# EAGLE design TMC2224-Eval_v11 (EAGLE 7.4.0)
CHECK_DATE: 24.01.14; DRAW_DATE: 27.01.14; PROJECT: DRV_Board_TMC261; REV: v1.0

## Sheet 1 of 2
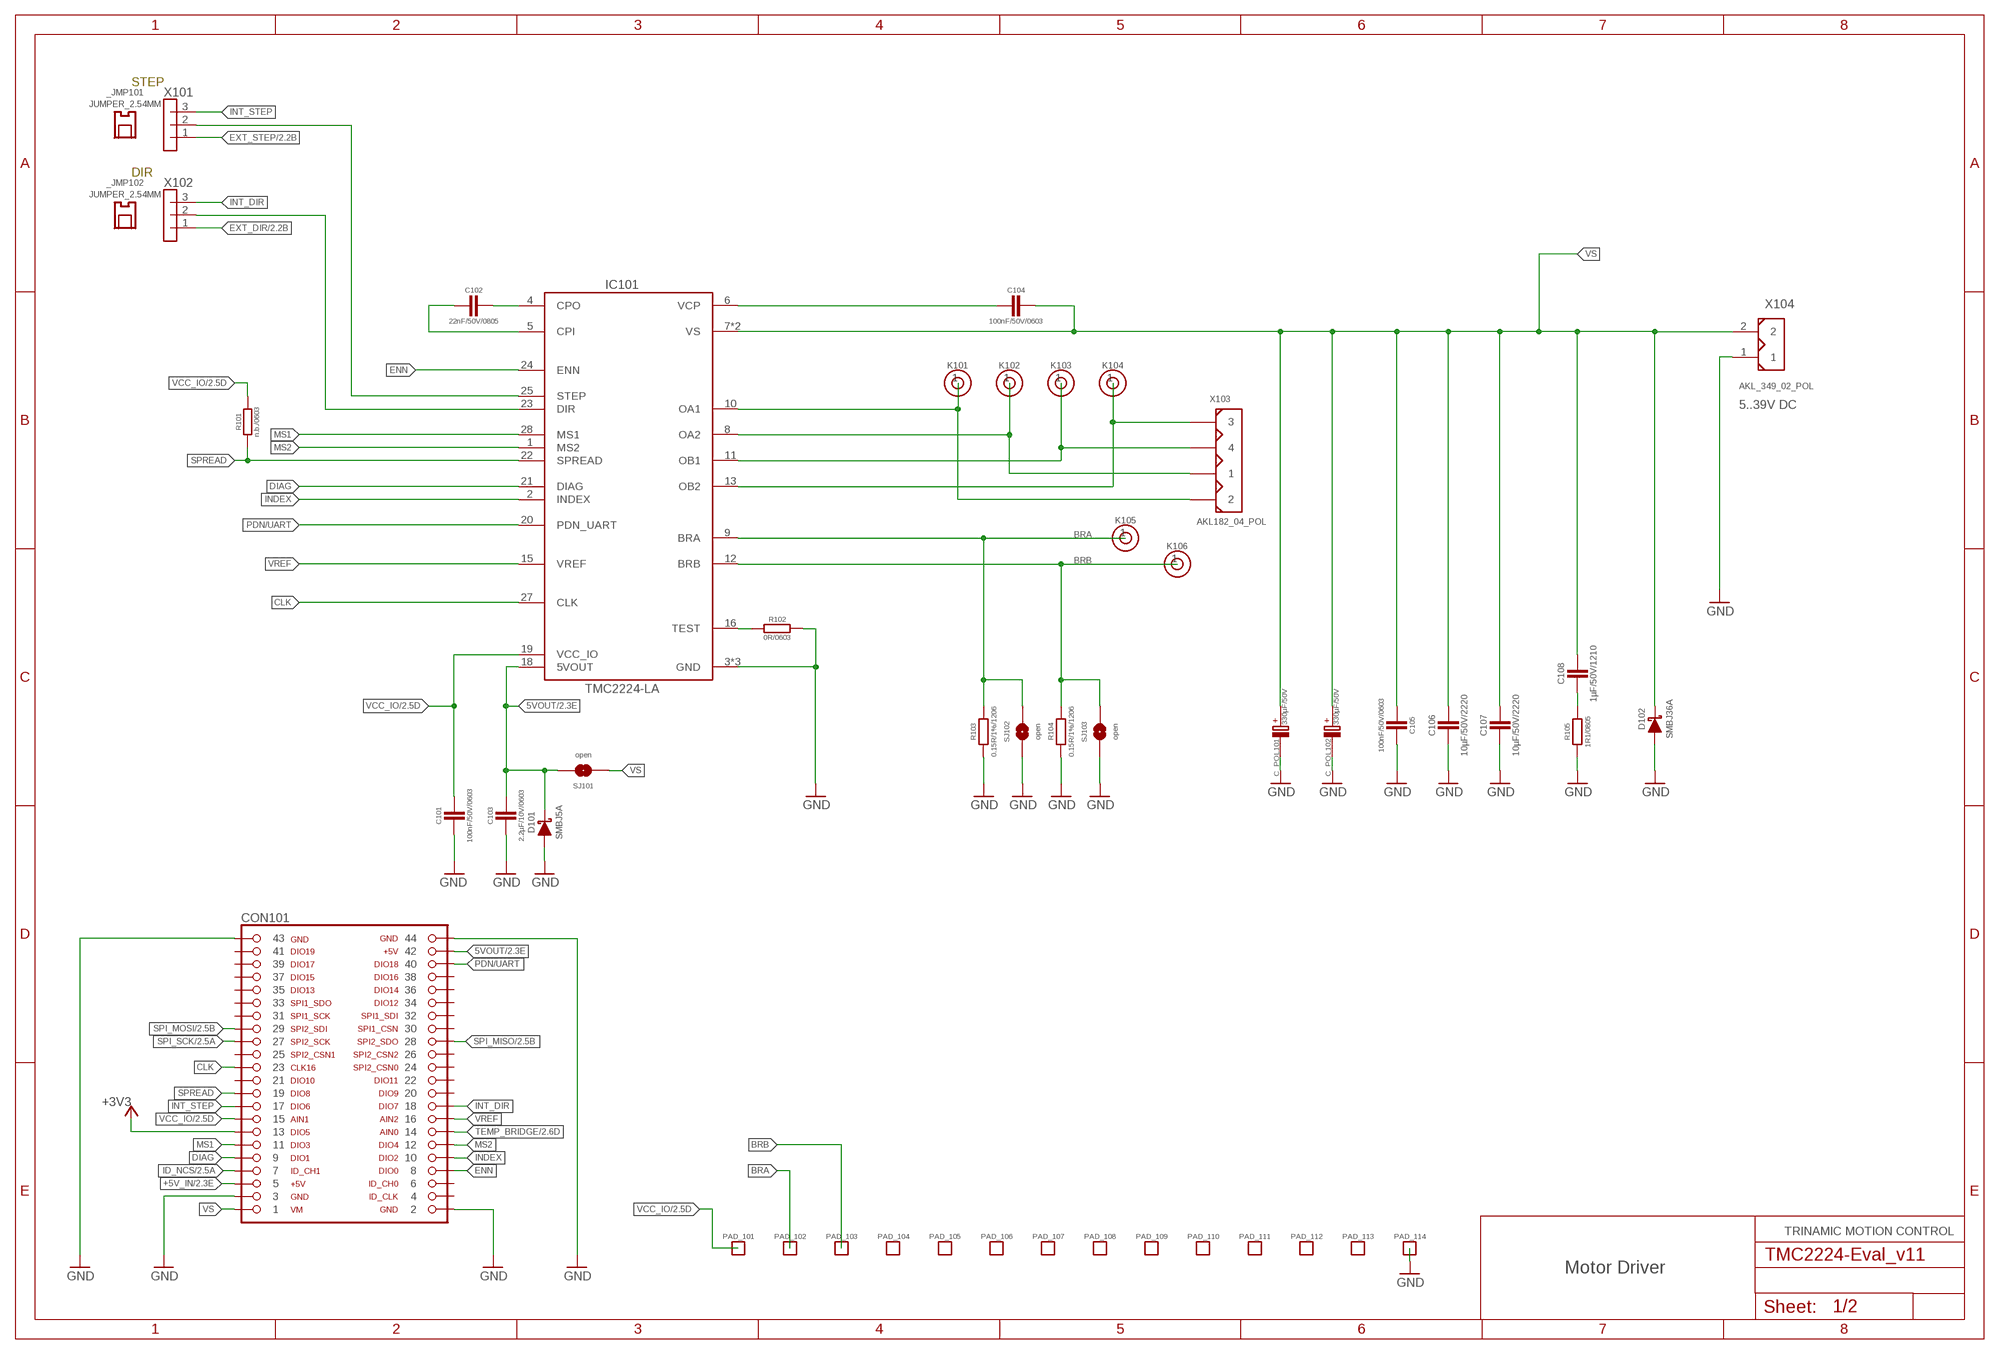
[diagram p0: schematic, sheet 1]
_JMP101 (JUMPER_2.54MM): ADGPN: 3044010200; DATASHEET: http://www.tme.eu/en/Document/d9e6fb6fc4dc34d59ba745016c42e7c7/jumper.pdf; MANUF-CODE-1: JUMPER-B; MANUFACTURER-1: Ninigi; PRICE: 0.11; SUPPLIER: TME; SUPPLIER-CODE: JUMPER-B
_JMP102 (JUMPER_2.54MM): ADGPN: 3044010200; DATASHEET: http://www.tme.eu/en/Document/d9e6fb6fc4dc34d59ba745016c42e7c7/jumper.pdf; MANUF-CODE-1: JUMPER-B; MANUFACTURER-1: Ninigi; PRICE: 0.11; SUPPLIER: TME; SUPPLIER-CODE: JUMPER-B

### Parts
C101  100nF/50V/0603  C0603  [_RC_0603]
C102  22nF/50V/0805  C0805  [_RC_0805]
C103  2.2µF/10V/0603  C0603  [_RC_0603]
C104  100nF/50V/0603  C0603  [_RC_0603]
C105  100nF/50V/0603  C0603  [_RC_0603]
C106  10µF/50V/2220  C2220  [C2220]
C107  10µF/50V/2220  C2220  [C2220]
C108  1µF/50V/1210  C1210  [C1210]
C_POL101  330µF/50V  C_POL5X10X17.5  [C_POL_RAD_THT_5X10]
C_POL102  330µF/50V  C_POL5X10X17.5  [C_POL_RAD_THT_5X10]
CON101  FEMALE_HEADER_SMD_2.54_44_PINSHORTPADS_HOLES  [FEMALE_HEADER_SMD_254_44_PIN_SHORTPADS_HOLES]
D101  SMBJ5A  SMBJ  [D_SMB]
D102  SMBJ36A  SMBJ48A  [D_SMB]
IC101  TMC2224-LA  [QFN28P]
K101  1PIN_1ROW  [1PIN_1ROW_THT]
K102  1PIN_1ROW  [1PIN_1ROW_THT]
K103  1PIN_1ROW  [1PIN_1ROW_THT]
K104  1PIN_1ROW  [1PIN_1ROW_THT]
K105  1PIN_1ROW  [1PIN_1ROW_THT]
K106  1PIN_1ROW  [1PIN_1ROW_THT]
PAD_101  PAD_ROUND  [PAD_R1.2]
PAD_102  PAD_ROUND  [PAD_R1.2]
PAD_103  PAD_ROUND  [PAD_R1.2]
PAD_104  PAD_ROUND  [PAD_R1.2]
PAD_105  PAD_ROUND  [PAD_R1.2]
PAD_106  PAD_ROUND  [PAD_R1.2]
PAD_107  PAD_ROUND  [PAD_R1.2]
PAD_108  PAD_ROUND  [PAD_R1.2]
PAD_109  PAD_ROUND  [PAD_R1.2]
PAD_110  PAD_ROUND  [PAD_R1.2]
PAD_111  PAD_ROUND  [PAD_R1.2]
PAD_112  PAD_ROUND  [PAD_R1.2]
PAD_113  PAD_ROUND  [PAD_R1.2]
PAD_114  PAD_ROUND  [PAD_R1.2]
R101  n.b./0603  0R/0603  [_RC_0603]
R102  0R/0603  [_RC_0603]
R103  0.15R/1%/1206  R1206  [_RC_1206]
R104  0.15R/1%/1206  R1206  [_RC_1206]
R105  1R1/0805  R0805  [_RC_0805]
SJ101  open  SJ  [_SJ_0402]
SJ102  open  SJ  [_SJ_0402]
SJ103  open  SJ  [_SJ_0402]
X101  3PIN_1ROWTHT  [3PIN_1ROM_2,54_THT]
X102  3PIN_1ROWTHT  [3PIN_1ROM_2,54_THT]
X103  AKL182_04_POL  [AKL169_04_POL]
X104  AKL_349_02_POL  [AKL349_02_POL]

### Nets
5VOUT: C103.P$1 CON101.42 D101.C IC101.18(5VOUT) SJ101.P$2 ; also sheet 2
+3V3: CON101.13 ; also sheet 2
+5V_IN: CON101.5 ; also sheet 2
BRA: IC101.9(BRA) K105.1 PAD_102.P$1 R103.P$2 SJ102.P$2
BRB: IC101.12(BRB) K106.1 PAD_103.P$1 R104.P$2 SJ103.P$2
CLK: CON101.23 IC101.27(CLK)
CPI: C102.P$2 IC101.5(CPI)
CPO: C102.P$1 IC101.4(CPO)
DIAG: CON101.9 IC101.21(DIAG)
DIR: IC101.23(DIR) X102.2
ENN: CON101.8 IC101.24(ENN)
EXT_DIR: X102.1 ; also sheet 2
EXT_STEP: X101.1 ; also sheet 2
GND: C101.P$2 C103.P$2 C105.P$2 C106.2 C107.2 C_POL101.- C_POL102.- CON101.2 CON101.3 CON101.43 CON101.44 D101.A D102.A IC101.3(GND) IC101.17(GND) IC101.PAD(GND) PAD_114.P$1 R102.P$2 R103.P$1 R104.P$1 R105.P$1 SJ102.P$1 SJ103.P$1 X104.1 ; also sheet 2
ID_NCS: CON101.7 ; also sheet 2
INDEX: CON101.10 IC101.2(INDEX)
INT_DIR: CON101.18 X102.3
INT_STEP: CON101.17 X101.3
MS1: CON101.11 IC101.28(MS1)
MS2: CON101.12 IC101.1(MS2)
N$2: C108.2 R105.P$2
OA1: IC101.10(OA1) K101.1 X103.1
OA2: IC101.8(OA2) K102.1 X103.2
OB1: IC101.11(OB1) K103.1 X103.3
OB2: IC101.13(OB2) K104.1 X103.4
PDN/UART: CON101.40 IC101.20(PDN_UART)
SPI_MISO: CON101.28 ; also sheet 2
SPI_MOSI: CON101.29 ; also sheet 2
SPI_SCK: CON101.27 ; also sheet 2
SPREAD: CON101.19 IC101.22(SPREAD) R101.P$1
STEP: IC101.25(STEP) X101.2
TEMP_BRIDGE: CON101.14 ; also sheet 2
TEST: IC101.16(TEST) R102.P$1
VCC_IO: C101.P$1 CON101.15 IC101.19(VCC_IO) PAD_101.P$1 R101.P$2 ; also sheet 2
VCP: C104.P$1 IC101.6(VCP)
VREF: CON101.16 IC101.15(VREF)
VS: C104.P$2 C105.P$1 C106.1 C107.1 C108.1 C_POL101.+ C_POL102.+ CON101.1 D102.C IC101.7(VS) IC101.14(VS) SJ101.P$1 X104.2
Unconnected: CON101.4 CON101.6 CON101.20 CON101.21 CON101.22 CON101.24 CON101.25 CON101.26 CON101.30 CON101.31 CON101.32 CON101.33 CON101.34 CON101.35 CON101.36 CON101.37 CON101.38 CON101.39 CON101.41 PAD_104.P$1 PAD_105.P$1 PAD_106.P$1 PAD_107.P$1 PAD_108.P$1 PAD_109.P$1 PAD_110.P$1 PAD_111.P$1 PAD_112.P$1 PAD_113.P$1

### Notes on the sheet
- STEP
- DIR
- 5..39V DC
- TRINAMIC MOTION CONTROL
- Motor Driver

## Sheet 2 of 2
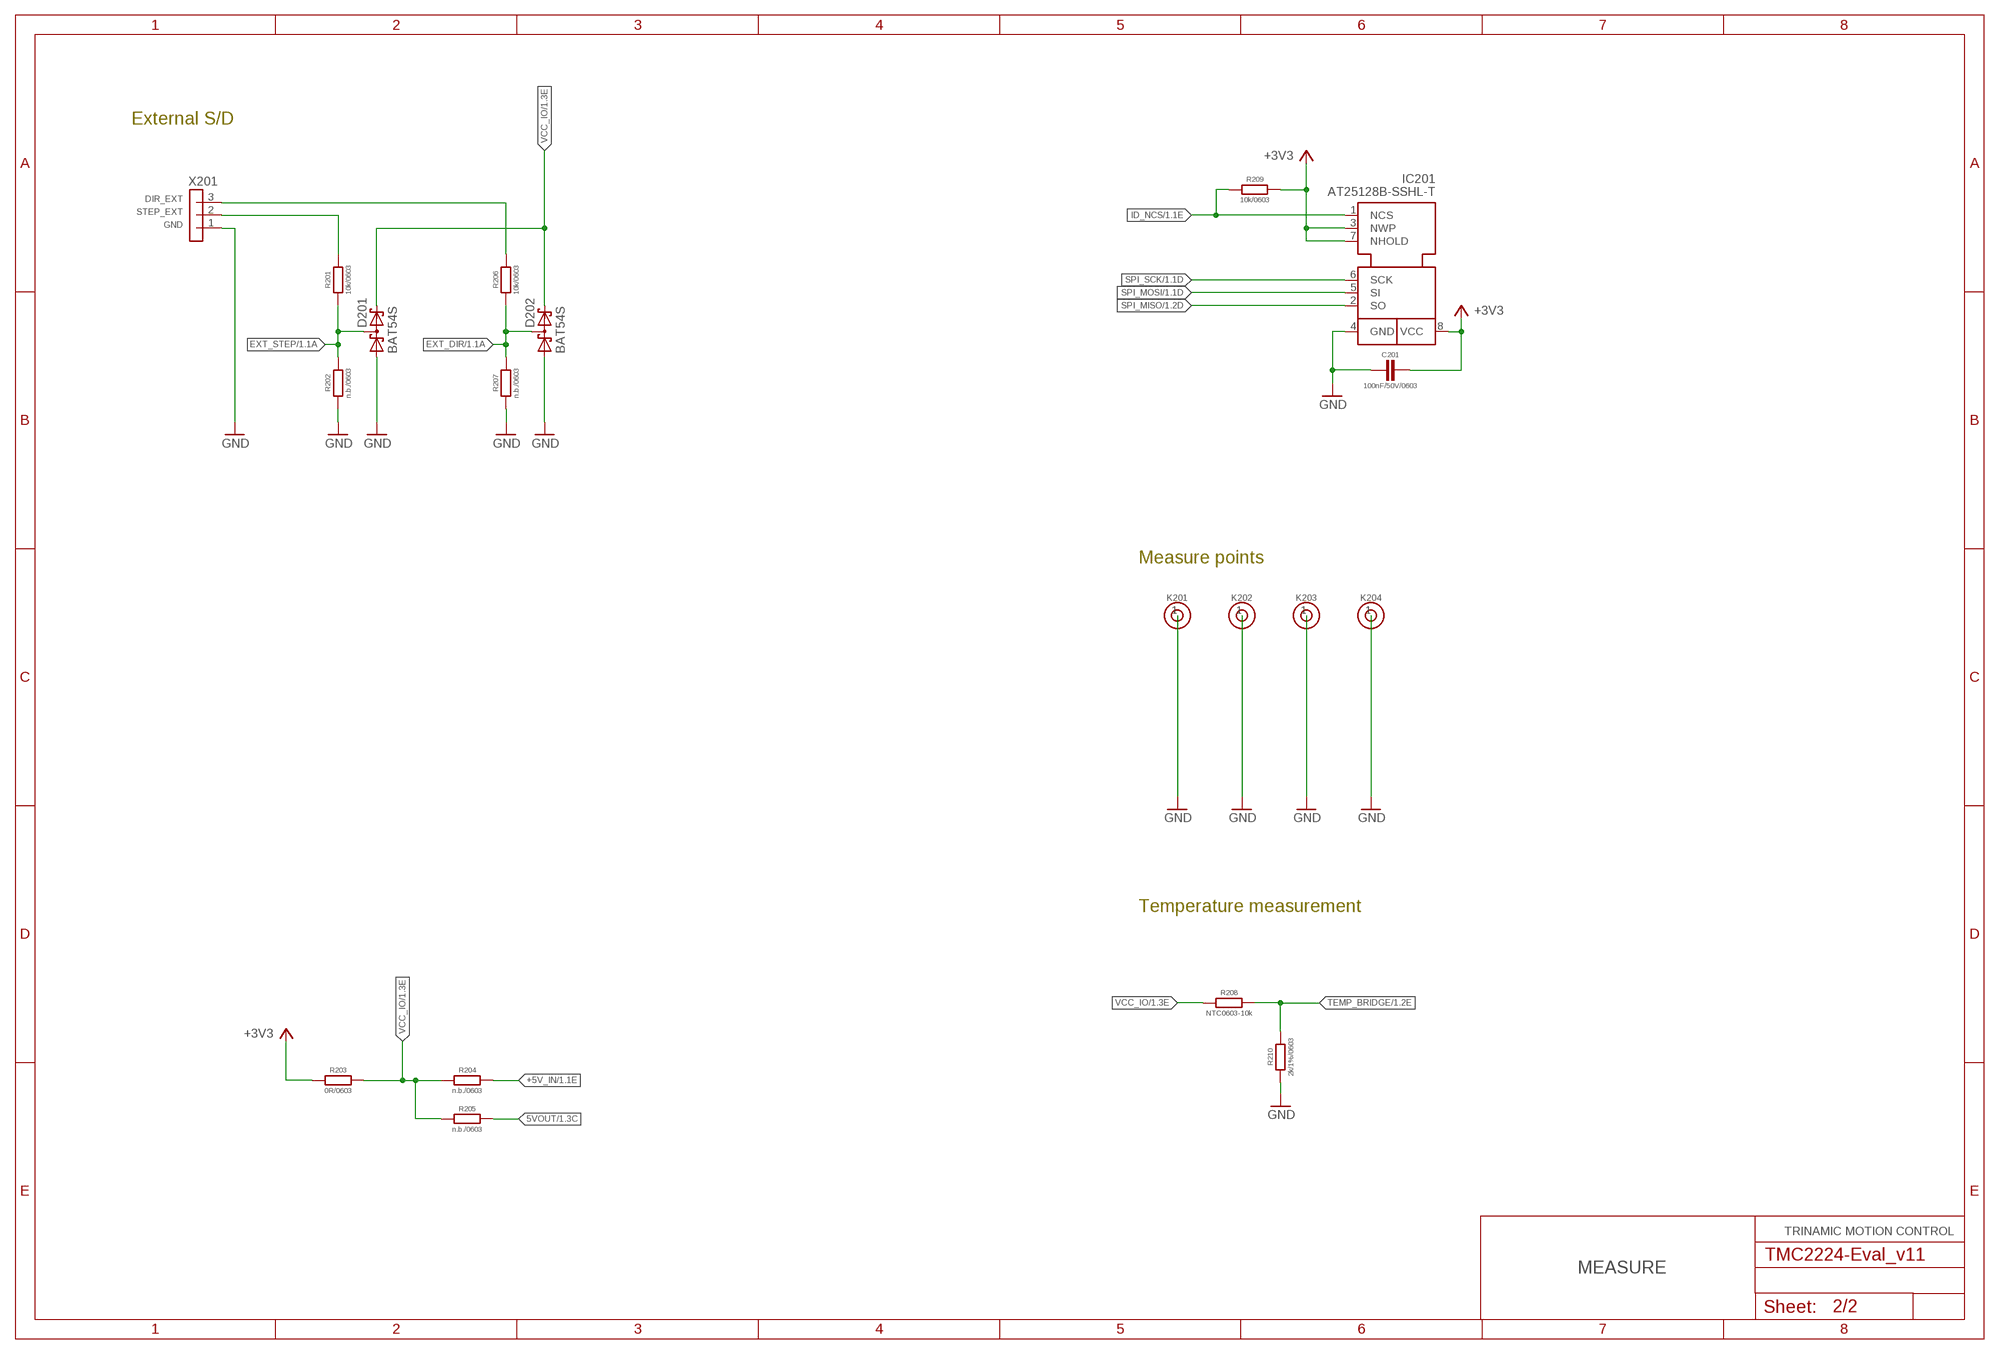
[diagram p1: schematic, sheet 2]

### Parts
C201  100nF/50V/0603  C0603  [_RC_0603]
D201  BAT54S  [SOT23]
D202  BAT54S  [SOT23]
IC201  AT25128B-SSHL-T  [SO8]
K201  1PIN_1ROW  [1PIN_1ROW_THT]
K202  1PIN_1ROW  [1PIN_1ROW_THT]
K203  1PIN_1ROW  [1PIN_1ROW_THT]
K204  1PIN_1ROW  [1PIN_1ROW_THT]
R201  10k/0603  R0603  [_RC_0603]
R202  n.b./0603  R0603  [_RC_0603]
R203  0R/0603  R0603  [_RC_0603]
R204  n.b./0603  R0603  [_RC_0603]
R205  n.b./0603  R0603  [_RC_0603]
R206  10k/0603  R0603  [_RC_0603]
R207  n.b./0603  R0603  [_RC_0603]
R208  NTC0603-10k  R0603  [_RC_0603]
R209  10k/0603  R0603  [_RC_0603]
R210  2k/1%/0603  R0603  [_RC_0603]
X201  3PIN_1ROWTHT  [3PIN_1ROM_2,54_THT]

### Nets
5VOUT: R205.P$2 ; also sheet 1
+3V3: C201.P$1 IC201.3(NWP) IC201.7(NHOLD) IC201.8(VCC) R203.P$1 R209.P$2 ; also sheet 1
+5V_IN: R204.P$2 ; also sheet 1
DIR_EXT: R206.P$2 X201.3
EXT_DIR: D202.3(C1A2) R206.P$1 R207.P$2 ; also sheet 1
EXT_STEP: D201.3(C1A2) R201.P$1 R202.P$2 ; also sheet 1
GND: C201.P$2 D201.1(A1) D202.1(A1) IC201.4(GND) K201.1 K202.1 K203.1 K204.1 R202.P$1 R207.P$1 R210.P$1 X201.1 ; also sheet 1
ID_NCS: IC201.1(NCS) R209.P$1 ; also sheet 1
SPI_MISO: IC201.2(SO) ; also sheet 1
SPI_MOSI: IC201.5(SI) ; also sheet 1
SPI_SCK: IC201.6(SCK) ; also sheet 1
STEP_EXT: R201.P$2 X201.2
TEMP_BRIDGE: R208.P$2 R210.P$2 ; also sheet 1
VCC_IO: D201.2(C2) D202.2(C2) R203.P$2 R204.P$1 R205.P$1 R208.P$1 ; also sheet 1

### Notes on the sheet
- External S/D
- Measure points
- Temperature measurement
- TRINAMIC MOTION CONTROL
- MEASURE

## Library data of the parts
C101-C105 C201 = TMC2208-Eval:C
C106 C107 = TMC2208-Eval:C*: Capacitor; OC_DIGIKEY: 445-7932-1-ND; SUPPLIER: DigiKey; SUPPLIER-CODE: 445-7932-1-ND
C108 = TMC2208-Eval:C*: Capacitor; OC_DIGIKEY: 1276-1811-1-ND; SUPPLIER: DigiKey; SUPPLIER-CODE: 1276-1811-1-ND
C_POL101 C_POL102 = TMC2208-Eval:C_POL; OC_DIGIKEY: 493-1343-ND; SUPPLIER: DigiKey; SUPPLIER-CODE: 493-1343-ND
CON101 = TMC2208-Eval:FEMALE_HEADER_SMD_2.54_44_PIN; SUPPLIER: MPE Garry; SUPPLIER-CODE: 098-3-044-1-NFX-YT0; SUPPLIER2: Samtec; SUPPLIER2-CODE: HLE-122-02-F-DV
D101 = TMC2208-Eval:SMBJ*: Surface Mount TRANSZORB Transient Voltage Suppressors 600W; MANUFACTURER: Bourns; OC_DIGIKEY: SMBJ5.0ABCT-ND; SUPPLIER: DigiKey; SUPPLIER-CODE: SMBJ5.0ABCT-ND
D102 = TMC2208-Eval:SMBJ*: Surface Mount TRANSZORB Transient Voltage Suppressors 600W; ADGPN: 4004048400; DATASHEET: http://www.bourns.com/data/global/pdfs/SMBJ.pdf; GEOMETRY_HEIGHT: 2.62mm; MANUFACTURER: Bourns; MANUFACTURER-CODE: SMBJ36A; OC_DIGIKEY: SMBJ36ABCT-ND; PRICE: 0,19; SUPPLIER: DigiKey; SUPPLIER-CODE: SMBJ36ABCT-ND
D201 D202 = TMC2208-Eval:BAT54S: SOT23, BAT54S, Double Schottky diode 30V 200mA Copied from diode.lbr and edited for Artec use 23-08-13 Pin connection corrected 2011-05-04 Source: Fairchild .. BAT54.pdf; ADGPN: 3522154300; DATASHEET: http://www.fairchildsemi.com/ds/BA/BAT54.pdf; MANUFACTURER: Fairchild; MANUFACTURER-CODE: BAT54S; OC_DIGIKEY: BAT54SFSCT-ND; PRICE: 0.12; SUPPLIER: DigiKey; SUPPLIER-CODE: BAT54SFSCT-ND
IC101 = TMC2224:TMC2224
IC201 = TMC2208-Eval:AT25128B; OC_DIGIKEY: AT25128B-SSHL-TCT-ND; SUPPLIER: DigiKey; SUPPLIER-CODE: AT25128B-SSHL-TCT-ND
K101-K106 K201-K204 = TMC2208-Eval:1PIN_1ROW
PAD_101-PAD_114 = TMC2208-Eval:PAD_ROUND
R101 R102 = TRI_R_0603:0R: Resistor (Jumper) 0603; MF: Panasonic; MPN: ERJ-3GEY0R00V; OC_DIGIKEY: P0.0GCT-ND; OR_SIMILAR: Yes; RATED_POWER: 1/10W
R103 R104 = TMC2208-Eval:R; OC_DIGIKEY: 408-1584-1-ND; SUPPLIER: DigiKey; SUPPLIER-CODE: 408-1584-1-ND
R105 = TMC2208-Eval:R; OC_DIGIKEY: RHM1.1KCT-ND; SUPPLIER-CODE: RHM1.1KCT-ND; SUPPLY: DigiKey
R201-R207 R209 R210 = TMC2208-Eval:R
R208 = TMC2208-Eval:R; OC_DIGIKEY: 445-174518-1-ND; SUPPLIER: DigiKey; SUPPLIER-CODE: 445-174518-1-ND
SJ101-SJ103 = TMC2208-Eval:SJ: SMD solder JUMPER
X101 X102 X201 = TMC2208-Eval:3PIN_1ROW
X103 = TMC2208-Eval:AKL182_04_POL; SUPPLIER: RIA CONNECT; SUPPLIER-CODE: 31182104; SUPPLIER2: Reichelt; SUPPLIER2-CODE: AKL 182-04
X104 = TMC2208-Eval:AKL_349_02_POL; SUPPLIER: RIA CONNECT; SUPPLIER-CODE: 31349102; SUPPLIER2: Reichelt; SUPPLIER2-CODE: AKL 349-02

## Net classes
0 default: clearance 0.2 mm
1 High Current: clearance 0.5 mm
2 VM: clearance 0.5 mm

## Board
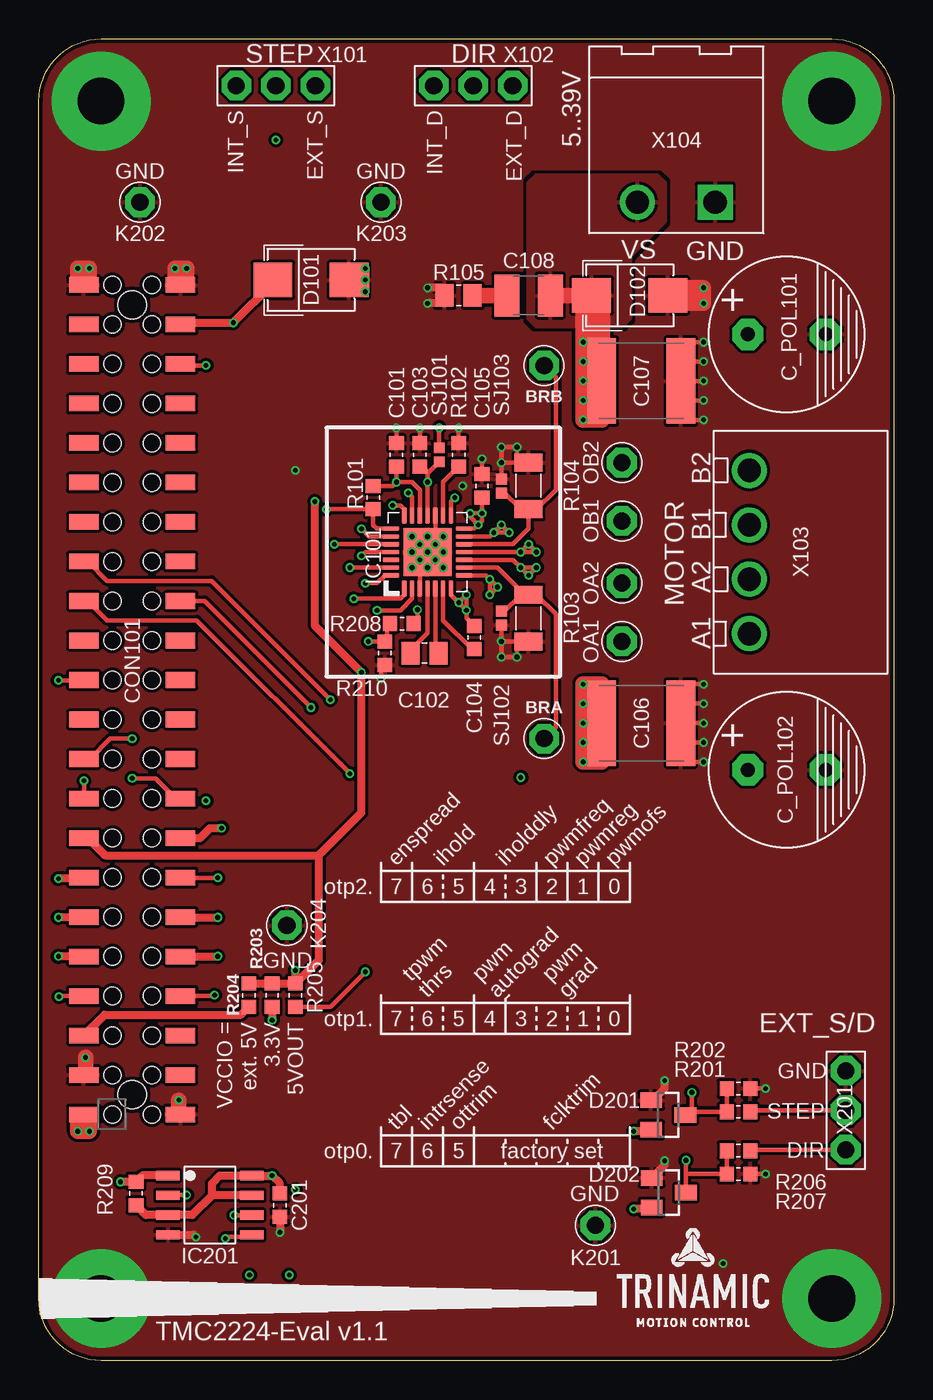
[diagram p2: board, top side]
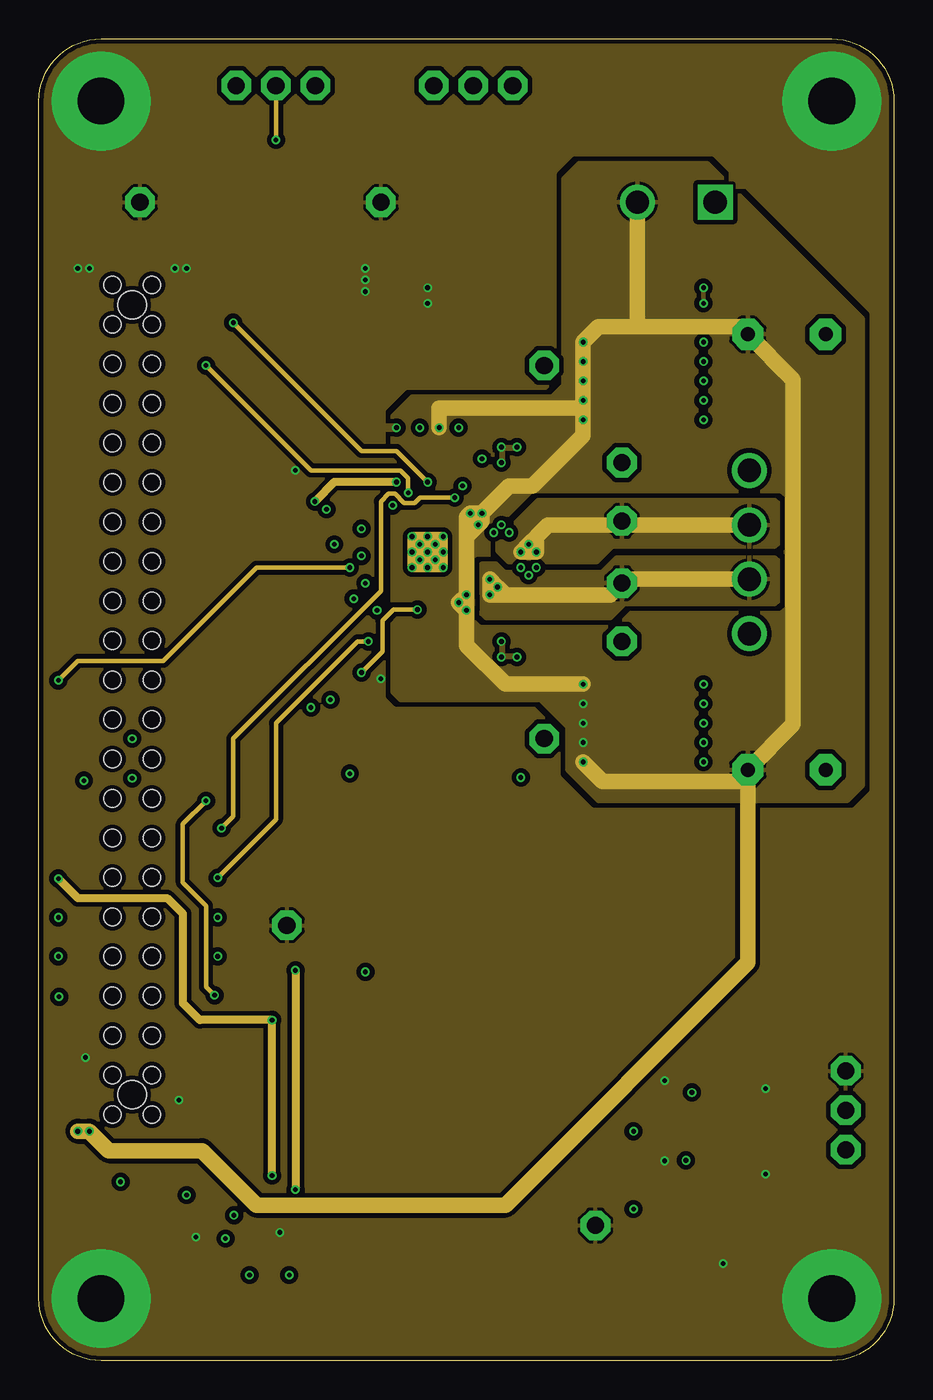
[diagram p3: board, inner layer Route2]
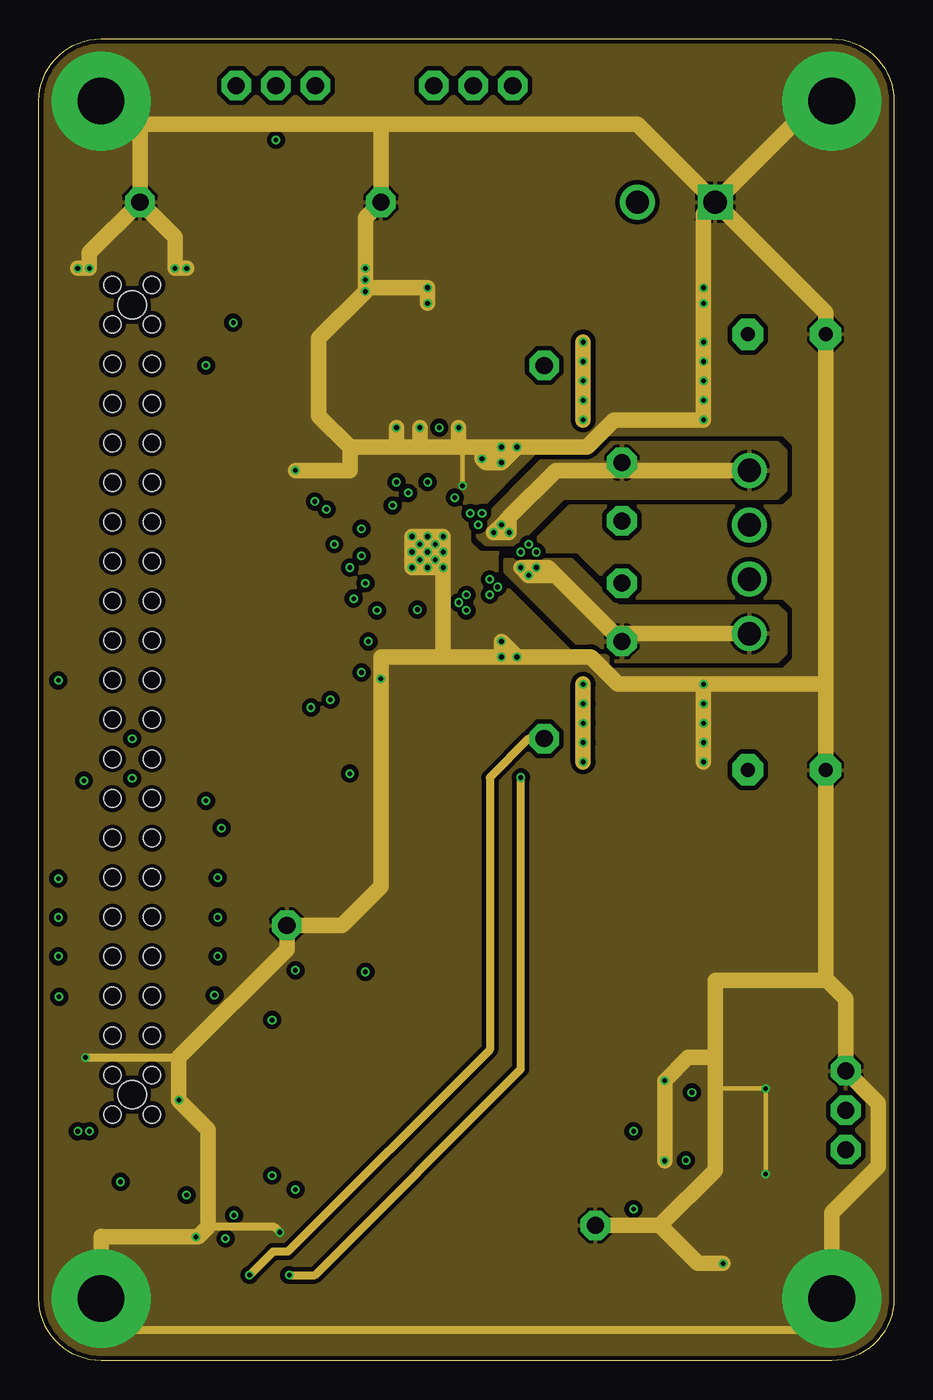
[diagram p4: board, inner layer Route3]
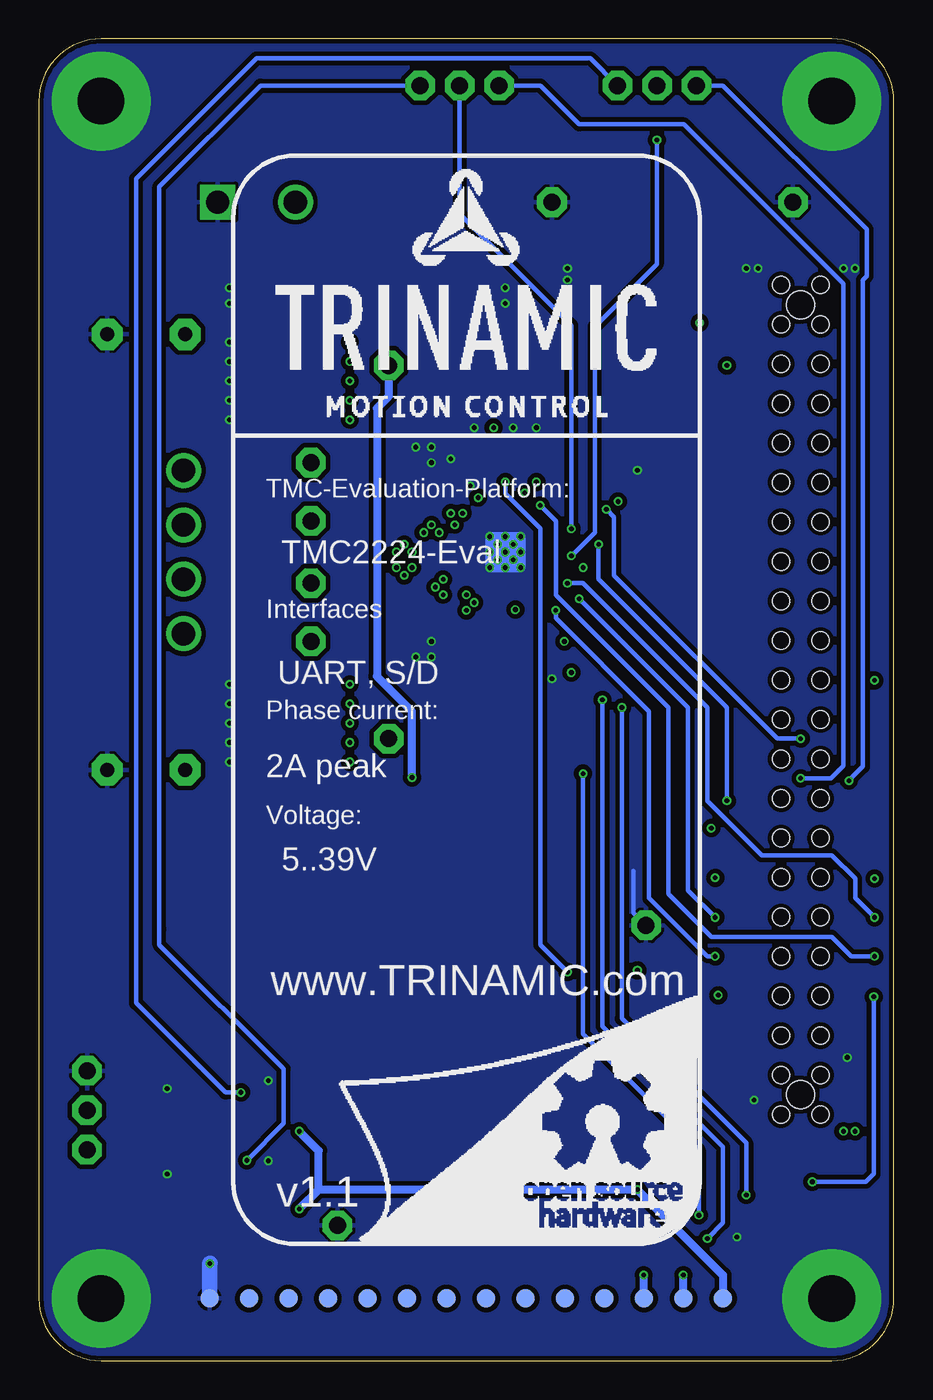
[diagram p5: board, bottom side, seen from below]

Size 55 x 85 mm. Coordinates in mm from the lower left corner, seen from the top.
Outline: 51,0 4,0 arc-90 0,4 0,81 arc-90 4,85 51,85 arc-90 55,81 55,4 arc-90 51,0
Copper layers (1+2*3+16): Top 0.018mm / dielectric 0.36mm / Route2 0.035mm / dielectric 0.71mm / Route3 0.035mm / dielectric 0.36mm / Bottom 0.018mm
Design rules "eC_4Layer_PClass6_BaseCopperO18-I35_eCDefault *": minimum track width 0.15mm, minimum drill 0.3mm, track to track 0.15mm, track to pad 0.15mm, pad to pad 0.15mm, via to via 0.15mm, smd to smd 0mil, copper to edge 0.25mm, drill to drill 0.33mm, minimum pad ring 0.175mm, minimum via ring 0.125mm, stop-mask expansion 0mil, vias tented up to drill 0.45mm, thermal gap 0.2mm

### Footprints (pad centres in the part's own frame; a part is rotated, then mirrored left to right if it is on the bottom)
_RC_0603 = smd 0.9 x 0.95: P$1 -0.75,0; P$2 0.75,0
_RC_0805 = smd 1.15 x 1.45: P$1 -0.9,0; P$2 0.9,0
C2220 = smd 1.85 x 5.5: 1 -2.55,0; 2 2.55,0
C1210 = smd 1.6 x 2.7: 1 -1.4,0; 2 1.4,0
C_POL_RAD_THT_5X10 = drill 0.9 pad 2 octagon: + 2.5,0; - -2.5,0
FEMALE_HEADER_SMD_254_44_PIN_SHORTPADS_HOLES = smd 1 x 1.9: 1 -26.67,3.11; 2 -26.67,-3.11; 3 -24.13,3.11; 4 -24.13,-3.11; 5 -21.59,3.11; 6 -21.59,-3.11; 7 -19.05,3.11; 8 -19.05,-3.11; 9 -16.51,3.11; 10 -16.51,-3.11; 11 -13.97,3.11; 12 -13.97,-3.11; 13 -11.43,3.11; 14 -11.43,-3.11; 15 -8.89,3.11; 16 -8.89,-3.11; 17 -6.35,3.11; 18 -6.35,-3.11; 19 -3.81,3.11; 20 -3.81,-3.11; 21 -1.27,3.11; 22 -1.27,-3.11; 23 1.27,3.11; 24 1.27,-3.11; 25 3.81,3.11; 26 3.81,-3.11; 27 6.35,3.11; 28 6.35,-3.11; 29 8.89,3.11; 30 8.89,-3.11; 31 11.43,3.11; 32 11.43,-3.11; 33 13.97,3.11; 34 13.97,-3.11; 35 16.51,3.11; 36 16.51,-3.11; 37 19.05,3.11; 38 19.05,-3.11; 39 21.59,3.11; 40 21.59,-3.11; 41 24.13,3.11; 42 24.13,-3.11; 43 26.67,3.11; 44 26.67,-3.11 | hole 1.8: -25.4,0; 25.4,0 | hole 1.1: -26.67,1.27; -24.13,1.27; -21.59,1.27; -19.05,1.27; -16.51,1.27; -13.97,1.27; -11.43,1.27; -8.89,1.27; -6.35,1.27; -3.81,1.27; -1.27,1.27; 1.27,1.27; 3.81,1.27; 6.35,1.27; 8.89,1.27; 11.43,1.27; 13.97,1.27; 16.51,1.27; 19.05,1.27; 21.59,1.27; 24.13,1.27; 26.67,1.27; -26.67,-1.27; -24.13,-1.27; -21.59,-1.27; -19.05,-1.27; -16.51,-1.27; -13.97,-1.27; -11.43,-1.27; -8.89,-1.27; -6.35,-1.27; -3.81,-1.27; -1.27,-1.27; 1.27,-1.27; 3.81,-1.27; 6.35,-1.27; 8.89,-1.27; 11.43,-1.27; 13.97,-1.27; 16.51,-1.27; 19.05,-1.27; 21.59,-1.27; 24.13,-1.27; 26.67,-1.27
D_SMB = smd 2.5 x 2.2: A 2.45,0; C -2.45,0
SOT23 = smd 1 x 1.4: 1 -0.95,-1.1; 2 0.95,-1.1; 3 0,1.1
QFN28P = smd 1.05 x 0.3: 1 -2.35,1.5; 2 -2.35,1; 3 -2.35,0.5; 4 -2.35,0; 5 -2.35,-0.5; 6 -2.35,-1; 7 -2.35,-1.5; 15 2.35,-1.5; 16 2.35,-1; 17 2.35,-0.5; 18 2.35,0; 19 2.35,0.5; 20 2.35,1; 21 2.35,1.5 | smd 0.3 x 1.05: 8 -1.5,-2.35; 9 -1,-2.35; 10 -0.5,-2.35; 11 0,-2.35; 12 0.5,-2.35; 13 1,-2.35; 14 1.5,-2.35; 22 1.5,2.35; 23 1,2.35; 24 0.5,2.35; 25 0,2.35; 26 -0.5,2.35; 27 -1,2.35; 28 -1.5,2.35 | smd 3.1 x 3.1: PAD 0,0
SO8 = smd 1.5 x 0.6: 1 -2.7,1.905; 2 -2.7,0.635; 3 -2.7,-0.635; 4 -2.7,-1.905; 5 2.7,-1.905; 6 2.7,-0.635; 7 2.7,0.635; 8 2.7,1.905
1PIN_1ROW_THT = drill 1.1 pad 1.9 octagon: 1 0,0
PAD_R1.2 = smd 1.2 x 1.2: P$1 0,0
_RC_1206 = smd 1.15 x 1.8: P$1 -1.5,0; P$2 1.5,0
_SJ_0402 = smd 0.7 x 0.7: P$1 -0.45,0; P$2 0.45,0
3PIN_1ROM_2,54_THT = drill 1.1 pad 1.9 octagon: 1 -2.54,0; 2 0,0; 3 2.54,0
AKL169_04_POL = drill 1.5: 1 -5.25,3.3; 2 -1.75,3.3; 3 1.75,3.3; 4 5.25,3.3
AKL349_02_POL = drill 1.5 square: 1 -2.5,4 | drill 1.5: 2 2.5,4

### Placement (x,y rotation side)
C101  23,58.25 90 top
C102  24.8,45.5 0 top
C103  24.5,58.25 90 top
C104  28,46.5 90 top
C105  28.5,56.25 90 top
C106  38.75,41 0 top
C107  38.75,63 0 top
C108  31.5,68.5 180 top
C201  15.5,10 270 top
C_POL101  48.1,66 180 top
C_POL102  48.1,38 180 top
CON101  6,42.5 90 top
D101  17.5,69.5 0 top
D102  38,68.5 0 top
D201  40.48,15.8 270 top
D202  40.52,10.8 270 top
IC101  25,52 90 top
IC201  11,10 0 top
K101  37.5,46.25 90 top
K102  37.5,50 90 top
K103  37.5,54 90 top
K104  37.5,57.75 90 top
K105  32.5,40 270 top
K106  32.5,64 0 top
K201  35.8,8.7 0 top
K202  6.5,74.5 0 top
K203  22,74.5 90 top
K204  15.95,28 180 top
PAD_101  11,4 270 bottom
PAD_102  13.54,4 270 bottom
PAD_103  16.08,4 270 bottom
PAD_104  18.62,4 270 bottom
PAD_105  21.16,4 270 bottom
PAD_106  23.7,4 270 bottom
PAD_107  26.24,4 270 bottom
PAD_108  28.78,4 270 bottom
PAD_109  31.32,4 270 bottom
PAD_110  33.86,4 270 bottom
PAD_111  36.4,4 270 bottom
PAD_112  38.94,4 270 bottom
PAD_113  41.48,4 270 bottom
PAD_114  44.02,4 270 bottom
R101  21.5,55.5 90 top
R102  27,58.25 90 top
R103  31.5,47.75 90 top
R104  31.5,56.25 270 top
R105  27,68.5 0 top
R201  45,16 0 top
R202  45,17.5 180 top
R203  15,23.5 90 top
R204  13.5,23.5 270 top
R205  16.5,23.5 270 top
R206  45,13.5 0 top
R207  45,12 180 top
R208  23.35,47.4 180 top
R209  6.25,10.75 270 top
R210  22.25,45.5 90 top
SJ101  25.75,58.25 270 top
SJ102  29.75,47.75 90 top
SJ103  29.75,56.25 270 top
U$1  [TMC_EVAL_RIGHT_BAR]  0,0 0 top
U$2  [TMC_EVAL_BACK_NO_DOCU]  55,0 0 bottom
X101  15.24,82 180 top
X102  27.94,82 180 top
X103  49,52 90 top
X104  41,78.5 180 top
X201  51.9,16.1 270 top

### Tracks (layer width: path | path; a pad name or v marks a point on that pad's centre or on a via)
5VOUT  (via drill 0.3)
  Top 0.3: SJ101.P$2 25.07,57.12 | 25.07,57.12 25,57.05 v25,56.5 IC101.18 | C103.P$1 24.7,57.5 25.07,57.12 | R205.P$2 18.75,22.75 v21,25
  Top 0.5: CON101.42 9.23,66.75 v12.5,66.75 15.05,69.3 D101.C
  Route2 0.3: v25,56.5 23,58.5 20.75,58.5 v12.5,66.75
  Bottom 0.3: v25,56.5 25,55.75 22.75,53.5 22.75,26.75 v21,25
+3V3  (via drill 0.3)
  Top 0.5: R209.P$2 6.88,9.37 IC201.3 9.87,9.37 11.13,10.63 | IC201.7 11.13,10.63 | 11.13,10.63 11.13,11.38 11.65,11.9 IC201.8 v15,11.9 15.5,11.4 C201.P$1 | CON101.13 2.82,31 v1.25,31 | R203.P$1 v15,21.9
  Route2 0.5: v1.25,31 2.5,29.75 8.25,29.75 9.25,28.75 9.25,23 10.35,21.9 v15,21.9 v15,11.9
+5V_IN
  Top 0.5: 2.31,20.91 CON101.5 4.23,22.25 13,22.25 R204.P$2
BRA  (via drill 0.3)
  Top 0.3: IC101.9 29.5,51 31.25,49.25 R103.P$2 | SJ102.P$2 29.95,48.2 31,49.25 R103.P$2 | K105.1 33.25,40.75 33.25,48 32,49.25 R103.P$2
  Route3 0.5: K105.1 31.5,40 29,37.5 29,20 16,7 15.05,7 v13.55,5.5
  Bottom 0.5: PAD_102.P$1 v13.54,5.49 v13.55,5.5
BRB  (via drill 0.3)
  Top 0.3: IC101.12 30.5,52.5 31.5,53.5 R104.P$2 | SJ103.P$2 29.95,55.8 31,54.75 R104.P$2 | K106.1 33.25,63.25 33.25,56 32,54.75 R104.P$2
  Route3 0.5: v16.1,5.5 17.75,5.5 31,18.75 v31,37.5
  Bottom 0.5: PAD_103.P$1 16.08,5.48 v16.1,5.5 | v31,37.5 31,41.75 33.25,44 33.25,61.25 32.5,62 K106.1
CLK  (via drill 0.3)
  Top 0.3: CON101.23 2.87,43.75 v1.25,43.75 | IC101.27 v20,51
  Top 0.5: CON101.23 3.02,43.77
  Route2 0.3: v1.25,43.75 2.5,45 8,45 14,51 v20,51
CPI
  Top 0.3: IC101.5 25.5,45.7 C102.P$2
CPO
  Top 0.3: IC101.4 25,46.8 23.9,45.7 C102.P$1
DIAG  (via drill 0.3)
  Top 0.3: IC101.21 23.5,54.75 23.25,55 v22.75,55
  Top 0.5: CON101.9 v1.25,26
  Bottom 0.3: v1.25,26 2.75,26 4,27.25 11.75,27.25 14.5,30 14.5,42 21.75,49.25 21.75,54 v22.75,55
DIR  (via drill 0.3)
  Top 0.3: IC101.23 21.25,53 v20.75,53.5
  Bottom 0.3: X102.2 27.94,73.75 20.75,66.56 v20.75,53.5
DIR_EXT
  Top 0.3: X201.3 45.81,13.56 R206.P$2
ENN  (via drill 0.3)
  Top 0.3: v11.3,23.5 11.25,23.45 CON101.8 | IC101.24 v19,52.5
  Route2 0.3: v11.3,23.5 10.75,24.05 10.75,29.25 9.25,30.75 9.25,34.5 v10.75,36
  Bottom 0.3: v10.75,36 10.75,42 19,50.25 v19,52.5
EXT_DIR  (via drill 0.3)
  Top 0.3: D202.3 41.62,12 | 41.62,12 v41.62,12.88 | R206.P$1 R207.P$2 41.62,12
  Bottom 0.3: X102.1 40.75,82 47.25,75.5 47.25,27.75 47.25,26.75 39.25,18.75 39.25,15.25 v41.62,12.88
EXT_STEP  (via drill 0.3)
  Top 0.3: v42,17.25 42,16.22 D201.3 41.78,16 R201.P$1 R202.P$2
  Bottom 0.3: v42,17.25 43,17.25 48.75,23 48.75,76 41,83.75 19.53,83.75 X101.1
GND  (via drill 0.3, 3 pad 6.35)
  Top 0.3: C107.2 v42.75,63 | C107.2 41.3,64.25 | 41.3,64.25 v42.75,64.25 | 41.3,64.25 41.3,65.5 v42.75,65.5 | C107.2 41.3,61.75 | 41.3,61.75 v42.75,61.75 | 41.3,61.75 41.3,60.5 v42.75,60.5 | C106.2 41.3,38.5 v42.75,38.5 | C106.2 41.3,39.75 v42.75,39.75 | C106.2 41.3,43.5 v42.75,43.5 | C106.2 41.3,42.25 v42.75,42.25 | C106.2 v42.75,41 | R202.P$1 v46.75,17.5 | R207.P$1 v46.75,12 | IC101.3 v24.5,51.5 | IC101.17 v25.5,52.5 | R104.P$1 30.75,57.75 | 30.75,57.75 v29.75,57.75 | v29.75,57.75 SJ103.P$1 | v29.75,57.75 v29.75,58.75 v30.75,58.75 30.75,57.75 | v29.75,46.25 v29.75,45.25 v30.75,45.25 30.75,46.25 R103.P$1 v29.75,46.25 | v29.75,46.25 SJ102.P$1 | C105.P$2 v28.5,58 | R102.P$2 v27,60 | C103.P$2 v24.5,60 | C101.P$2 v23,60 | R210.P$1 22,44.75 v22,43.85
  Top 0.406: IC101.PAD 25,52.05 | 25,52.05 v25,53 | 25,52.05 24.55,52.5 v24.5,52.5 v24,53 | IC101.PAD 25.05,52.05 | 25.05,52.05 v25.5,52.5 v26,53 | IC101.PAD v26,52 | IC101.PAD v24,52 | v24,51 v24.5,51.5 IC101.PAD | IC101.PAD v25,51 | 25.05,52.05 26,51.1 v26,51 | IC101.PAD v25.5,51.5
  Top 0.5: v21,69.5 v21,70.25 19.54,70.25 19.54,68.75 v21,68.75 v21,69.5 | v25,69 26.05,69 26.05,68 | 26.05,68 v25,68 | D201.1 39.5,16.75 40.25,17.5 v40.25,18 | D202.1 40.25,12.58 v40.25,12.85 | 26.05,68 26.1,68 R105.P$1 | C201.P$2 v15.5,8.25 | D101.A v21,69.5 | IC201.4 9.96,8.1 v10.1,7.95
  Top 1: 9.5,69.5 9.5,69.17 CON101.44 8.75,69.17 v8.75,70.25 | 9.5,69.5 v9.5,70.25 v8.75,70.25 | v8.75,70.25 8.75,69.5 9.5,69.5 | 3.25,69.75 3.25,69.17 CON101.43 2.5,69.17 v2.5,70.25 | 3.25,69.75 v3.25,70.25 v2.5,70.25 | v2.5,70.25 2.5,69.75 3.25,69.75 | CON101.3 3,18.37 v3,19.5 | CON101.2 9,15.83 v9,16.75 | D102.A 40.45,69 v42.75,69 v42.75,68 40.45,68 D102.A
  Route2 0.6: v24,53 v25,53 v26,53 v26,52 v26,51 v25,51 v24,51 v24,52 v24,53 | v24,53 v24.5,52.5 | v24.5,52.5 v25.5,52.5 | v25.5,52.5 v25.5,51.5 | v25.5,51.5 v24.5,51.5 | v24.5,51.5 v24.5,52.5 | v24.5,52.5 IC101.PAD | IC101.PAD v25.5,51.5 | v25.5,52.5 IC101.PAD | IC101.PAD v24.5,51.5
  Route3 0.3: v46.75,12 v46.75,17.5 43.5,17.5 | v27.25,56.25 27.25,58.75
  Route3 0.5: v3,19.5 9,19.5 | v4,4 6,2 49,2 v51,4 | v15.5,8.25 15.15,8.6 10.9,8.6
  Route3 1: 50.6,43.5 C_POL102.- 50.6,24.55 | 50.6,43.5 C_POL101.- 50.6,67.4 X104.1 | X104.1 42.75,73.75 v42.75,69 v42.75,68 v42.75,65.5 v42.75,64.25 v42.75,63 v42.75,61.75 v42.75,60.5 37,60.5 35.25,58.75 v30.75,58.75 | v42.75,43.5 50.6,43.5 | v42.75,38.5 v42.75,39.75 v42.75,41 v42.75,42.25 v42.75,43.5 | X104.1 50,81 v51,81 | v4,81 5.5,79.5 6.5,79.5 | 6.5,79.5 22,79.5 | 22,79.5 38.5,79.5 X104.1 | v30.75,58.75 v29.75,58.75 | v29.75,58.75 29,58.75 | 29,58.75 28.75,58.75 | 28.75,58.75 27.25,58.75 | 27.25,58.75 24.5,58.75 | 24.5,58.75 23.05,58.75 | 23.05,58.75 20,58.75 | 22,79.5 K203.1 21,73.5 v21,70.25 v21,69.5 21,69 | v25,68 v25,69 21,69 | 21,69 v21,68.75 18,65.75 18,60.75 20,58.75 | K202.1 8.75,72.25 v8.75,70.25 v9.5,70.25 | v2.5,70.25 v3.25,70.25 3.25,71.25 K202.1 | K202.1 6.5,79.5 | 20,58.75 20,57.25 v16.5,57.25 | v26,52 v26,53 v25,53 v24,53 v24,52 v24,51 v25,51 | v25,51 v26,51 | v26,51 v26,52 | v26,52 v25.5,51.5 v24.5,51.5 v24.5,52.5 v25.5,52.5 v26,52 | 50.6,24.55 50.6,24.46 43.5,24.46 43.5,19.5 | 50.6,24.55 51.9,23.25 X201.1 54,16.54 54,12.5 51,9.5 v51,4 | 43.5,19.5 43.5,17.5 43.5,12.25 39.95,8.7 | 43.5,19.5 41.75,19.5 v40.25,18 v40.25,12.85 | K201.1 39.95,8.7 | v44,6.25 42.4,6.25 39.95,8.7 | v4,4 4,7.95 | 4,7.95 4,8 | 4,7.95 v10.1,7.95 10.25,7.95 10.9,8.6 10.9,14.85 v9,16.75 9,19.5 15.95,26.45 K204.1 19.5,28 22,30.5 v22,43.85 22,45.25 26,45.25 | v25,51 IC101.PAD | v30.75,45.25 v29.75,45.25 | v29.75,45.25 v29.75,46.25 v30.75,45.25 | v29.75,45.25 26,45.25 | v30.75,45.25 35.5,45.25 37.25,43.5 v42.75,43.5 | v29.75,57.75 29.75,57.85 | v29.75,57.75 v29.75,58.75 | 28.75,58.75 28.5,58.5 v28.5,58 28.75,57.75 v29.75,57.75
  Route3 1: v27,60 R102.P$2 27.25,58.75 | v24.5,60 24.5,58.75 | v23,60 23,58.8 23.05,58.75 | v29.75,57.75 29,58.5 29,58.75 | v29.75,57.75 v30.75,58.75 | v26,51 26,45.25
  Bottom 0.3: K204.1 16.75,28.8 16.75,31.5
  Bottom 0.6: v24,53 v26,53 v26,51 v24,51 v24,53 | v24,53 v24.5,52.5 | v24.5,52.5 v25.5,52.5 v25.5,51.5 v24.5,51.5 v24.5,52.5 | v24.5,52.5 IC101.PAD
  Bottom 1: PAD_114.P$1 44.02,6.23 v44,6.25
  other vias: 25,52
  pour Route2 (isolate 0.3, rank 6): 0,-0.09 0,85 55,85 55,0
  pour Route3 (isolate 0.3, rank 6): 55,85 0,85 0,-0.09 55,0
  pour Top (isolate 0.2, rank 6): 55,85 0,85 0,-0.09 55,0
  pour Bottom (isolate 0.3, rank 2): 0,0 55,0 55,85 0,85
ID_NCS  (via drill 0.3)
  Top 0.3: v1.3,23.4 1.35,23.45 CON101.7
  Top 0.5: IC201.1 6.66,11.9 R209.P$1 v5.25,11.5
  Bottom 0.3: v1.3,23.4 1.3,12 1.8,11.5 v5.25,11.5
INDEX  (via drill 0.3)
  Top 0.3: IC101.2 24,49 23.25,48.25 v21.75,48.25
  Top 0.5: CON101.10 v11.5,26
  Bottom 0.3: v11.5,26 12,26 15.75,29.75 15.75,41.75 21.75,47.75 v21.75,48.25
INT_DIR  (via drill 0.3)
  Top 0.3: v6,37.45 7.5,37.45 8.8,36.15 CON101.18
  Bottom 0.3: v6,37.45 4.05,37.45 3.25,38.25 3.25,69.25 13.5,79.5 20.25,79.5 22.75,82 X102.3
INT_STEP  (via drill 0.3)
  Top 0.3: v2.9,37.3 CON101.17
  Bottom 0.3: v2.9,37.3 2,38.2 2,69.5 1.75,69.75 1.75,72.75 11,82 X101.3
MS1  (via drill 0.3)
  Top 0.3: IC101.28 22.25,50.5 21.75,50 v21,50
  Top 0.5: CON101.11 2.86,28.5 v1.25,28.5
  Bottom 0.3: v1.25,28.5 2.5,29.75 2.5,31 4,32.5 8.5,32.5 12,36 12,42 20,50 v21,50
MS2  (via drill 0.3)
  Top 0.3: IC101.1 23.5,49.25 23.25,49 v20.25,49
  Top 0.5: CON101.12 9.14,28.5 v11.5,28.5
  Bottom 0.3: v11.5,28.5 13.25,30.25 13.25,42 v20.25,49
N$2
  Top 0.3: R105.P$2 27.95,68.5
  Top 1: 27.95,68.5 30,68.5 C108.2
OA1  (via drill 0.3)
  Top 0.3: IC101.10 30.5,51.5 v31,51 | v31,51 v31.5,50.5 v32,51 v31,51
  Route3 1: v32,51 v31,51 v31.5,50.5 | v31.5,50.5 v32,51 | v31.5,50.5 33.25,50.5 | 33.25,50.5 37,46.75 37.75,46.75 | v32,51 32.75,51 33.25,50.5 | X103.1 37.75,46.75 | K101.1 37.5,46.5 37.75,46.75
  pour Route3 (isolate 0.3, rank 4): 47.5,48.5 48,48 48,45.5 47.5,45 35.75,45 30,50.75 30,51.5 34.25,51.5 37.25,48.5
OA2  (via drill 0.3)
  Top 0.3: IC101.8 28.75,50.5 v29,50.25 | v29,50.25 v29.5,49.75 v29,49.25 v29,50.25
  Route2 1: X103.2 37.75,50.25 K102.1 36.75,49.25 32,49.25 30,49.25 | 30,49.25 29.05,49.25 | 29.05,49.25 v29,49.25 | 29.05,49.25 29,49.3 v29,50.25 v29.5,49.75 30,49.25
  pour Route2 (isolate 0.3, rank 4): 47.35,51.65 37.15,51.65 36.2,50.7 29.95,50.7 29.4,51.25 28.5,51.25 28.25,51 28.25,48.25 28.75,47.75 36.75,47.75 37.65,48.65 47.35,48.65 47.55,48.85 47.55,51.45
OB1  (via drill 0.3)
  Top 0.3: IC101.11 v31,52 | v31,52 v31.5,52.5 v32,52 v31,52
  Route2 1: X103.3 37.5,53.75 | 37.5,53.75 K103.1 | v32,52 v31,52 v31.5,52.5 | v31.5,52.5 v32,52 | v31.5,52.5 32,53 | 37.5,53.75 32.75,53.75 32.25,53.25 32,53 | v32,52 32,53
  pour Route2 (isolate 0.3, rank 4): 47.35,55.35 32.1,55.35 29.5,52.75 29.5,52.05 30.2,51.35 35.9,51.35 36.9,52.35 47.35,52.35 47.55,52.55 47.55,55.15
OB2  (via drill 0.3)
  Top 0.3: IC101.13 29,53 v29.25,53.25 | v29.25,53.25 v29.75,53.75 v30.25,53.25 v29.25,53.25
  Route3 1: X103.4 37.6,57.25 | 37.6,57.25 33.25,57.25 30.25,54.25 | 30.25,54.25 v29.75,53.75 v29.25,53.25 v30.25,53.25 30.25,54.25 | K104.1 37.5,57.35 37.6,57.25
  pour Route3 (isolate 0.3, rank 4): 47.5,55.5 48,56 48,58.5 47.5,59 36.5,59 35.5,58 32.5,58 28.25,53.75 28.25,53 28.75,52.5 30.75,52.5 33.75,55.5
PDN/UART  (via drill 0.3)
  Top 0.3: CON101.40 9.2,64 v10.75,64 | IC101.20 24,55.55 v23.75,55.8
  Route2 0.3: v23.75,55.8 23.75,56.75 23.25,57.25 17.5,57.25 v10.75,64
SPI_MISO  (via drill 0.3)
  Top 0.3: IC201.2 8.31,10.65 v9.5,10.65 | CON101.28 10.65,48.85 v17.5,42
  Bottom 0.3: v17.5,42 17.5,22 9.5,14 v9.5,10.65
SPI_MOSI  (via drill 0.3)
  Top 0.3: IC201.5 13.55,7.95 12.1,7.95 v12,7.85 | CON101.29 3.16,51.39 4.4,50.15 11.1,50.15 v18.75,42.5
  Bottom 0.3: v18.75,42.5 18.75,21.5 11,13.75 11,8.85 v12,7.85
SPI_SCK  (via drill 0.3)
  Top 0.3: IC201.6 13.69,9.35 v12.55,9.35 | CON101.27 3.15,48.85 4.4,47.6 10.15,47.6 v20,37.75
  Bottom 0.3: v20,37.75 20,21 12.55,13.55 v12.55,9.35
SPREAD  (via drill 0.3)
  Top 0.3: IC101.22 21.75,53.5 21.5,53.75 R101.P$1 v18.5,54.75 | v6,40 4.6,40 3.29,38.69 CON101.19
  Bottom 0.3: v18.5,54.75 18,54.25 18,50.5 7.5,40 v6,40
STEP  (via drill 0.3)
  Top 0.3: IC101.25 21,52 v20.75,51.75
  Route2 0.3: X101.2 v15.25,78.5
  Bottom 0.3: v15.25,78.5 15.25,70.5 19.25,66.5 19.25,53.25 v20.75,51.75
STEP_EXT
  Top 0.3: X201.2 45.85,16.1 R201.P$2
TEMP_BRIDGE  (via drill 0.3)
  Top 0.3: R208.P$2 22.4,47.4 22.4,46.25 R210.P$2 v21.2,46.25 | v11.5,31.05 9.13,31.05 CON101.14
  Route2 0.3: v21.2,46.25 20.5,46.25 15.25,41 15.25,34.8 v11.5,31.05
TEST
  Top 0.3: IC101.16 26,56.5 R102.P$1
VCC_IO  (via drill 0.3)
  Top 0.3: C101.P$1 v23,56.5 | v23,56.5 24,56.5 24.5,56 IC101.19 | R101.P$2 22.75,56.25 v23,56.5 | R208.P$1 24.35,47.4 v24.35,48.3
  Top 0.5: D201.2 39.28,14.75 v38.25,14.75 | D202.2 39.32,9.75 v38.25,9.75 | R204.P$1 R203.P$2 R205.P$1 | CON101.15 3.14,33.61 4.25,32.5 18,32.5 | v17.75,55.25 17.75,47.25 v20.75,44.25 20.75,35.25 18,32.5 | 18,32.5 18,25.75 R205.P$1 | R205.P$1 v16.5,25.1
  Route2 0.3: v24.35,48.3 22.8,48.3 22.1,47.6 22.1,45.6 v20.75,44.25
  Route2 0.5: v23,56.5 19,56.5 v17.75,55.25 | v16.5,25.1 v16.5,11
  Bottom 0.5: 37,11 v16.5,11 11,5.5 PAD_101.P$1 | 37,11 v38.25,9.75 | 37,11 37,13.5 v38.25,14.75
VCP
  Top 0.3: IC101.6 26,47.6 27.85,45.75 C104.P$1
VREF  (via drill 0.3)
  Top 0.3: IC101.15 26.5,55.25 v26.75,55.5
  Top 0.5: CON101.16 10.36,33.61 11,34.25 v11.75,34.25
  Route2 0.3: v26.75,55.5 24.5,55.5 24.15,55.15 23.5,55.15 22.9,55.75 22.5,55.75 22,55.25 22,49.5 12.5,40 12.5,35 v11.75,34.25
VS  (via drill 0.3)
  Top 0.3: C107.1 36.2,61.75 | IC101.14 28,53.5 v28.25,53.75 | v28.25,53.75 28.5,54 v28.5,54.5 | v28.5,54.5 C105.P$1 | v28.5,54.5 v27.75,54.5 27.75,54.25 v28.25,53.75 | C104.P$2 27.5,47.75 v27.5,48.25 | v27.5,48.25 v27,48.75 | v27,48.75 26.5,49.25 IC101.7 | v27,48.75 v27.5,49.25 v27.5,48.25 | SJ101.P$1 v25.75,60
  Top 0.5: C108.1 33,68.5
  Top 1: C107.1 v35,63 | C107.1 36.2,65.5 v35,65.5 | C107.1 36.2,64.25 v35,64.25 | 36.2,61.75 v35,61.75 | C107.1 36.2,60.5 v35,60.5 v35,61.75 | 36.2,42.25 36.2,43.5 v35,43.5 v35,42.25 | C106.1 36.2,42.25 | 36.2,42.25 v35,42.25 | C106.1 v35,41 | C106.1 36.2,39.75 | 36.2,39.75 v35,39.75 | 36.2,39.75 36.2,38.5 v35,38.5 v35,39.75 | v35,61.75 v35,63 | v35,63 v35,64.25 | v35,64.25 v35,65.5 | v35,42.25 v35,41 | v35,41 v35,39.75 | CON101.1 2.89,14.75 v2.5,14.75 | v2.5,14.75 2.5,15.75 3.25,15.75 v3.25,14.75 v2.5,14.75 | 33,68.5 35.5,68.5 | 35.5,68.5 D102.C | v35,65.5 35,67.95 D102.C | D102.C 36.25,67.8 36.25,65 35.5,65 35.5,68.5
  Route2 1: 35,61.25 v35,61.75 v35,63 v35,64.25 v35,65.5 36,66.5 38.5,66.5 | 35,61.25 v35,60.5 35,59.5 31.75,56.25 30.25,56.25 v28.5,54.5 | C_POL102.+ 44.85,37.25 | 44.85,37.25 36.25,37.25 v35,38.5 | 38.5,66.5 45.1,66.5 C_POL101.+ 48.5,63.1 48.5,40.9 C_POL102.+ | X104.2 38.5,66.5 | v2.5,14.75 v3.25,14.75 4.5,13.5 10.5,13.5 14,10 30,10 45.6,25.6 45.6,37.25 | 45.6,37.25 C_POL102.+ | 45.6,37.25 44.85,37.25 | v25.75,60 25.75,61.25 35,61.25 | v28.25,53.75 27.75,54.25 v27.75,54.5 | v27.75,54.5 v28.5,54.5 | v28.5,54.5 28.5,54 v28.25,53.75 | v27.5,48.25 v27,48.75 v27.5,49.25 | v27.5,49.25 v27.5,48.25 | v27.5,49.25 27.5,53 | 27.5,53 27.5,54.25 v27.75,54.5 | v28.25,53.75 27.5,53 | v35,43.5 30,43.5 27.5,46 v27.5,48.25
  Route3 1: v35,38.5 v35,39.75 v35,41 v35,42.25 v35,43.5 | v35,65.5 v35,64.25 v35,63 v35,61.75 v35,60.5
  pour Route2 (isolate 0.3, rank 5): 43,77 34.75,77 33.75,76 33.75,62.75 33,62 24,62 22.75,60.75 22.75,43 23.25,42.5 32.25,42.5 34,40.75 34,38 36,36 52,36 53,37 53,67
  pour Top (isolate 0.3, rank 5): 37.5,66.5 32,66.5 31.5,67 31.5,75.75 32,76.25 39.75,76.25 40.25,75.75 40.25,73.25 38,71 38,67

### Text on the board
Top: Top
Route2: Inner1
Route3: Inner2
Bottom: Bottom
tPlace: STEP | DIR | INT_S | EXT_S | INT_D | EXT_D | 5..39V | GND | GND | VS | GND | BRB | Silkscreen Top | OB2 | B2 | OB1 | B1 | MOTOR | OA2 | A2 | A1 | OA1 | BRA | enspread | ihold | iholddly | pwmfreq | pwmreg | pwmofs | otp2. | 7 | 6 | 5 | 4 | 3 | 2 | 1 | 0 | GND | tpwm / thrs | pwm / autograd | pwm / grad | VCCIO = | ext. 5V | 3.3V | 5VOUT | otp1. | 7 | 6 | 5 | 4 | 3 | 2 | 1 | 0 | EXT_S/D | GND | STEP | tbl | intrsense | ottrim | fclktrim | otp0. | 7 | 6 | 5 | factory set | DIR | GND | TMC2224-Eval v1.1
bPlace: TMC-Evaluation-Platform: | Silkscreen Bottom | TMC2224-Eval | Interfaces | UART, S/D | Phase current: | 2A peak | Voltage: | 5..39V | v1.1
